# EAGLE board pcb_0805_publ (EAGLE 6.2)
DATA: 28-08-2013; WERSJA: 1.1+SMD / FINAL
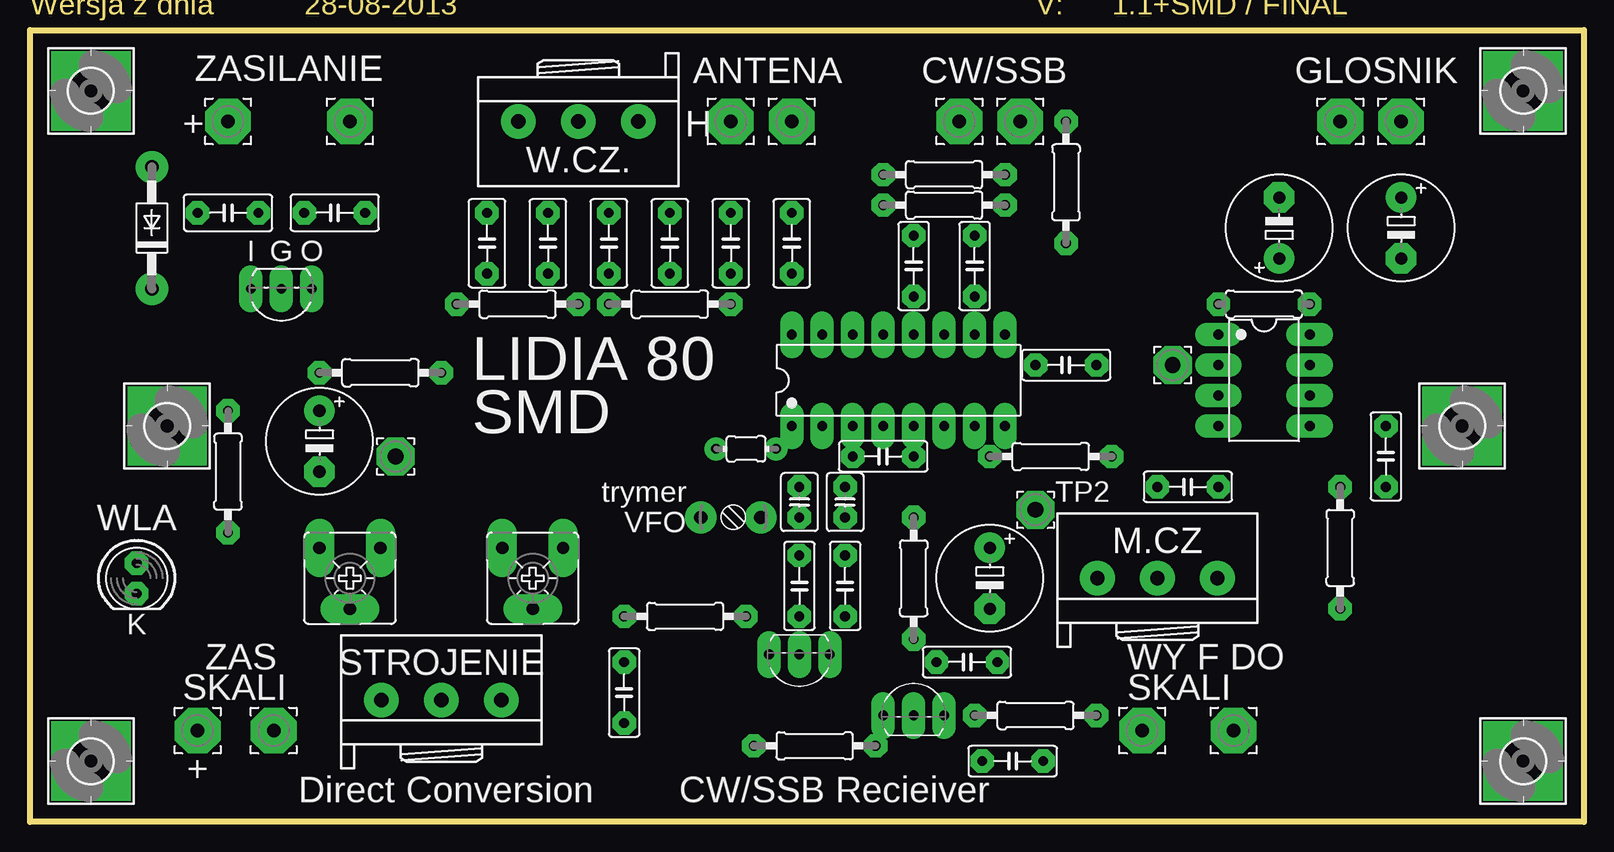
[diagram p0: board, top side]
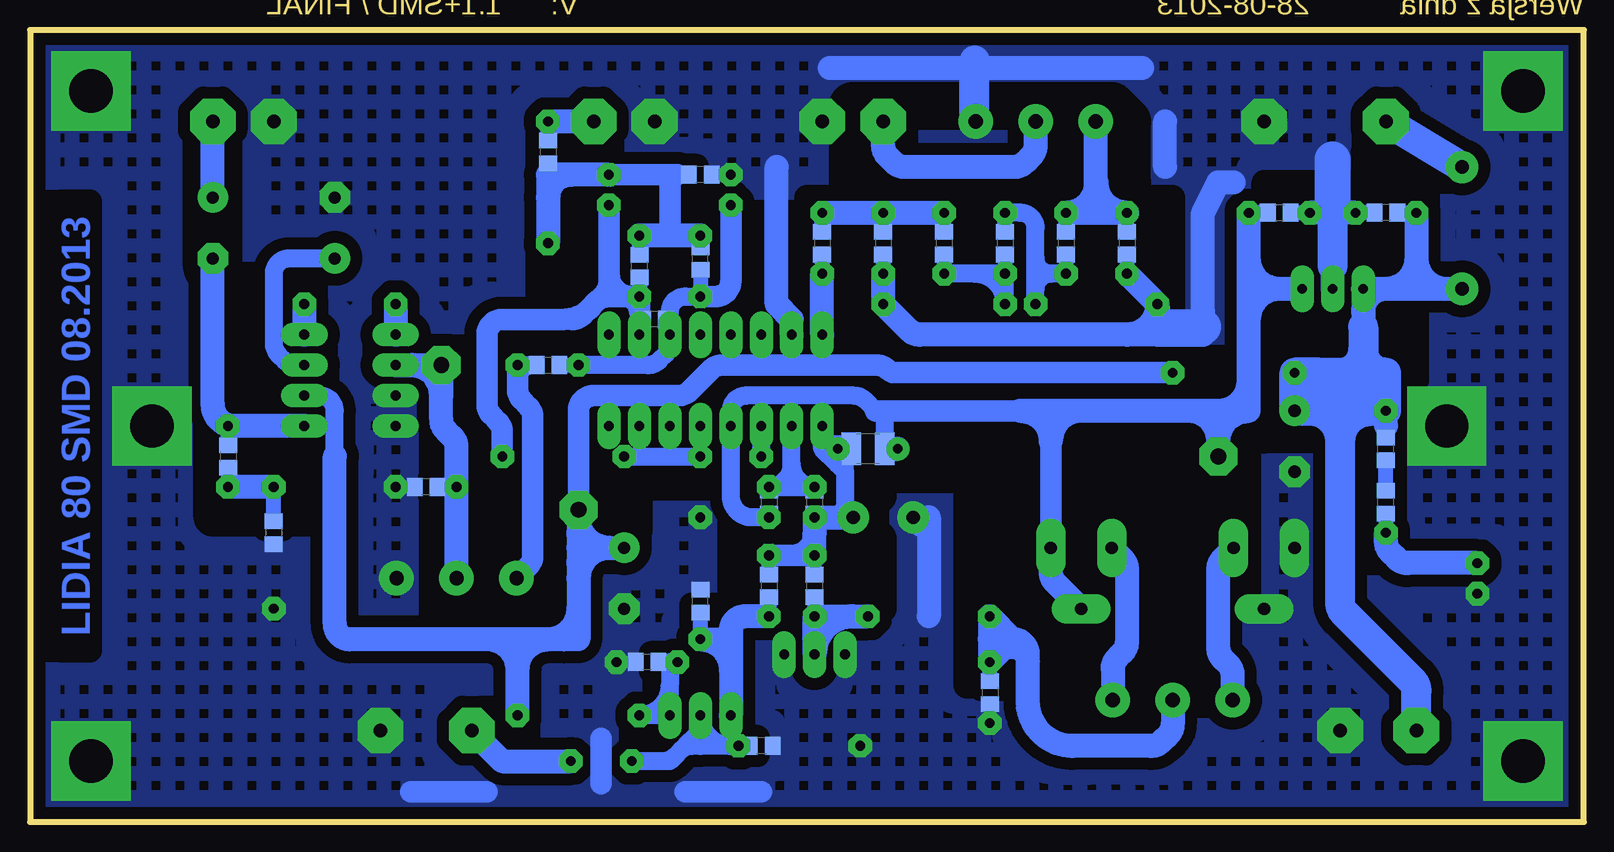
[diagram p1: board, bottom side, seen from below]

Size 129.54 x 66.04 mm. Coordinates in mm from the lower left corner, seen from the top.
Outline: 0,0 0,66.04 129.54,66.04 129.54,0 0,0
Copper layers (1*16): Top 0mil / dielectric 1.5mm / Bottom 0.035mm
Design rules: minimum track width 10mil, minimum drill 24mil, track to track 8mil, track to pad 8mil, pad to pad 8mil, via to via 8mil, smd to smd 8mil, copper to edge 5mil, drill to drill 5mil, minimum pad ring 0.1mm, minimum via ring 8mil, stop-mask expansion 10mil, vias tented up to drill 0mil, thermal gap 19mil
bRestrict: area 34.3,39.4 to 69.8,52.1; area 14,31.8 to 26.7,53.3; 28 lines

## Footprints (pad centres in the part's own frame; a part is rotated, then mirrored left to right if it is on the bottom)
3,81/1,1 = drill 1.118 pad 3.81 octagon: 1 0,0
E5-8,5 = drill 1.016 pad 2.54: + -2.54,0 | drill 1.016 pad 2.54 octagon: - 2.54,0
C050-030X075 = drill 0.813 octagon: 1 -2.54,0; 2 2.54,0
C050-025X075 = drill 0.813 octagon: 1 -2.54,0; 2 2.54,0
3050-504 = drill 1.1: 1 -2.5,0; 2 2.5,0
C025-030X050 = drill 0.813 octagon: 1 -1.27,0; 2 1.27,0
DO41-10 = drill 1.118: A 5.08,0; C -5.08,0
TO92- = drill 0.813 long: 1 2.54,0; 2 0,0; 3 -2.54,0
3,6-PAD-SQUARE = drill 3.6 pad 5.842 square: B3,6 0,0
C0805 = smd 1.3 x 1.5: 1 -0.95,0; 2 0.95,0
0207/7 = drill 0.813 octagon: 1 -3.81,0; 2 3.81,0
LAP02KR = drill 0.8 pad 1.3: 1 -2.5,0; 2 2.5,0
C1210 = smd 1.6 x 2.7: 1 -1.4,0; 2 1.4,0
0207/10 = drill 0.813 octagon: 1 -5.08,0; 2 5.08,0
LED5MM = drill 0.813 octagon: A -1.27,0; K 1.27,0
3RP/1610N = drill 1.2 pad 2.184: 1 -5,0; 2 0,0; 3 5,0
CA6V = drill 1.016 long: A -2.54,-2.54; E 2.54,-2.54; S 0,2.54
3,17/1,3 = drill 1.321 pad 3.175 octagon: 1 0,0
TO92-LINE = drill 0.813 long: 1 2.54,0; 2 0,0; 3 -2.54,0
DIL16 = drill 0.813 long: 1 -8.89,-3.81; 2 -6.35,-3.81; 3 -3.81,-3.81; 4 -1.27,-3.81; 5 1.27,-3.81; 6 3.81,-3.81; 7 6.35,-3.81; 8 8.89,-3.81; 9 8.89,3.81; 10 6.35,3.81; 11 3.81,3.81; 12 1.27,3.81; 13 -1.27,3.81; 14 -3.81,3.81; 15 -6.35,3.81; 16 -8.89,3.81
DIL08 = drill 0.813 long: 1 -3.81,-3.81; 2 -1.27,-3.81; 3 1.27,-3.81; 4 3.81,-3.81; 5 3.81,3.81; 6 1.27,3.81; 7 -1.27,3.81; 8 -3.81,3.81

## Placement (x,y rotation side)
+  [3,81/1,1]  16.51,58.42 0 top
+1  [3,81/1,1]  26.67,58.42 0 top
A_GND  [3,81/1,1]  63.5,58.42 0 top
C1  100uF  [E5-8,5]  24.13,31.75 270 top
C2  100µF  [E5-8,5]  80.01,20.32 270 top
C3  100µF  [E5-8,5]  104.14,49.53 90 top
C4  100µF  [E5-8,5]  114.3,49.53 270 top
C5  680pF  [C050-030X075]  38.1,48.26 90 top
C6  270pF  [C050-030X075]  43.18,48.26 90 top
C7  10pF  [C050-030X075]  48.26,48.26 90 top
C8  270pF  [C050-030X075]  53.34,48.26 90 top
C9  680pF  [C050-030X075]  58.42,48.26 90 top
C10  1nF  [C050-030X075]  63.5,48.26 90 top
C11  47nF  [C050-025X075]  73.66,46.35 90 top
C12  47nF  [C050-025X075]  78.74,46.35 90 top
C13  100nF  [C050-025X075]  86.36,38.1 180 top
C14  47nF  [C050-025X075]  96.52,27.94 180 top
C15  100nF  [C050-025X075]  113.03,30.48 90 top
C16  10nF  [C050-025X075]  71.12,30.48 180 top
C17  10-50pF  [3050-504]  58.42,25.4 0 top
C18  100nF  [C050-030X075]  25.4,50.8 180 top
C19  100nF  [C050-030X075]  16.51,50.8 0 top
C20  100nF  [C050-025X075]  49.53,10.79 270 top
C21  100pF  [C025-030X050]  64.14,26.67 270 top
C22  2*100pF  [C025-030X050]  67.94,26.67 270 top
C23  10nF  [C050-025X075]  64.14,19.68 270 top
C24  2,7-10pF  [C050-025X075]  67.94,19.68 270 top
C25  10nF  [C050-025X075]  81.92,5.08 0 top
C26  100nF  [C050-025X075]  78.11,13.34 0 top
CW/SSB  [3,81/1,1]  82.55,58.42 0 top
CW/SSB_GND  [3,81/1,1]  77.47,58.42 0 top
CW/SSB_GND1  [3,81/1,1]  92.71,7.62 0 top
CW/SSB_GND2  [3,81/1,1]  100.33,7.62 0 top
CW/SSB_GND3  [3,81/1,1]  20.32,7.62 0 top
CW/SSB_GND4  [3,81/1,1]  13.97,7.62 0 top
D1  1N4007  [DO41-10]  10.16,49.53 90 top
D2*  BB104G  [TO92-]  64.14,13.97 180 top
E$1  [3,6-PAD-SQUARE]  5.08,60.96 0 top
E$2  [3,6-PAD-SQUARE]  11.43,33.02 0 top
E$3  [3,6-PAD-SQUARE]  5.08,5.08 0 top
E$4  [3,6-PAD-SQUARE]  124.46,5.08 0 top
E$5  [3,6-PAD-SQUARE]  119.38,33.02 0 top
E$6  [3,6-PAD-SQUARE]  124.46,60.96 0 top
E$7  100nF  [C0805]  16.51,50.8 180 bottom
E$8  100nF  [C0805]  25.4,50.8 0 bottom
E$9  100nF  [C0805]  86.36,38.1 0 bottom
E$10  100nF  [C0805]  49.53,10.79 270 bottom
E$11  100nF  [C0805]  113.03,30.48 270 bottom
E$12  22Ω  [C0805]  109.22,24.13 270 bottom
E$13  47Ω  [C0805]  86.36,55.88 270 bottom
E$14  47Ω  [C0805]  73.66,53.98 180 bottom
E$15  gain  [0207/7]  102.87,43.18 0 top
E$16  10µH  [LAP02KR]  59.69,31.11 0 top
E$21  [ICON_PIN1_B]  63.5,34.92 0 top
E$22  [ICON_PIN1_B]  100.97,40.64 0 top
E$23  47nF  [C0805]  96.52,27.94 180 bottom
E$24  2,7-10pF  [C0805]  67.94,19.68 270 bottom
E$25  10nF  [C0805]  64.14,19.68 270 bottom
E$26  100pF  [C0805]  64.14,26.67 270 bottom
E$27  100pF  [C0805]  67.94,26.67 270 bottom
E$28  100nF  [C0805]  78.11,13.34 180 bottom
E$29  1MΩ  [C0805]  73.66,18.41 90 bottom
E$30  1kΩ  [C0805]  16.51,26.67 90 bottom
E$31  1kΩ  [C0805]  16.51,31.11 90 bottom
E$33  270pF  [C0805]  43.18,48.26 270 bottom
E$34  10pF  [C0805]  48.26,48.26 270 bottom
E$35  270pF  [C0805]  53.34,48.26 270 bottom
E$36  1nF  [C0805]  63.5,48.26 270 bottom
E$37  100kΩ  [C0805]  77.47,41.91 180 bottom
E$38  47nF  [C0805]  73.66,46.99 90 bottom
E$39  47nF  [C0805]  78.74,46.35 90 bottom
E$40  1kΩ  [C0805]  68.58,6.35 180 bottom
E$41  680pF  [C0805]  38.1,48.26 270 bottom
E$42  680pF  [C0805]  58.42,48.26 270 bottom
GLOGND  [3,81/1,1]  109.22,58.42 0 top
GLOSNIK  GLOSNIK  [3,81/1,1]  114.3,58.42 0 top
L1*  10µH  [C1210]  59.69,31.11 180 bottom
L2  10µH  [0207/10]  40.64,43.18 0 top
L3  10µH  [0207/10]  53.34,43.18 0 top
L4  100µH  [0207/10]  83.82,8.89 0 top
LED1  WLA  [LED5MM]  8.89,20.32 270 top
POT1  1kΩ  [3RP/1610N]  45.72,58.42 180 top
POT2  50kΩ  [3RP/1610N]  93.98,20.32 0 top
POT3  10kΩ  [3RP/1610N]  34.29,10.16 0 top
PR1  10kΩ  [CA6V]  26.67,20.32 180 top
PR2  10kΩ  [CA6V]  41.91,20.32 180 top
R1  2,2kΩ  [0207/10]  16.51,29.21 90 top
R2  220Ω  [0207/10]  29.21,37.47 0 top
R3  47Ω  [0207/10]  76.2,53.98 0 top
R4  100kΩ  [0207/10]  76.2,51.44 0 top
R5  47Ω  [0207/10]  86.36,53.34 90 top
R6  22Ω  [0207/10]  109.22,22.86 270 top
R7  7,5kΩ  [0207/10]  85.09,30.48 0 top
R8  100kΩ  [0207/10]  54.61,17.14 180 top
R9  1MΩ  [0207/10]  73.66,20.32 270 top
R10  1kΩ  [0207/10]  65.41,6.35 180 top
SGN  [3,81/1,1]  58.42,58.42 0 top
T1  BF245  [TO92-]  73.66,8.89 0 top
TP1  [3,17/1,3]  30.48,30.48 0 top
TP2  [3,17/1,3]  83.82,26.04 0 top
TP3  [3,17/1,3]  95.25,38.1 0 top
US1  78L08  [TO92-LINE]  20.95,44.45 180 top
US2  MC3361C  [DIL16]  72.39,36.83 0 top
US3  LM368N  [DIL08]  102.87,36.83 270 top

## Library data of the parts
+ +1 A_GND CW/SSB CW/SSB_GND CW/SSB_GND1-CW/SSB_GND4 GLOGND GLOSNIK SGN TP1-TP3 = wirepad
C1-C16 C18-C26 E$7-E$16 E$23-E$31 E$33-E$42 L1* L2-L4 R1-R10 = rcl
C17 = c-trimm
D1 = diode
D2* = transistor-npn
E$1-E$6 = holes
E$21 E$22 = dicons
LED1 = led
POT1-POT3 PR1 PR2 = pot
T1 = transistor-fet
US1 = transistor-small-signal
US2 US3 = ic-package

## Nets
GND: +1.1 A_GND.1 C1.- C2.- C3.- C5.1 C9.1 C14.1 C17.1 C18.2 C19.2 C20.2 C26.2 CW/SSB_GND2.1 CW/SSB_GND3.1 CW/SSB_GND.1 D2*.1 D2*.3 E$1.B3,6 E$2.B3,6 E$3.B3,6 E$4.B3,6 E$5.B3,6 E$6.B3,6 E$7.2 E$8.2 E$10.2 E$12.2 E$14.1 E$23.2 E$28.2 E$29.2 E$40.1 E$41.2 E$42.2 GLOGND.1 L2.1 L3.2 LED1.K POT1.1 POT2.3 PR1.E PR1.S R3.1 R6.2 R9.1 R10.2 US1.2 US2.15 US3.3 US3.4
S$1: POT1.2 SGN.1
S$2: C5.2 C6.2 E$33.1 E$41.1 POT1.3
S$3: C10.1 E$36.2 US2.16
S$4: C21.1 C22.1 US2.2
S$5: +.1 D1.A
S$6: C1.+ C19.1 CW/SSB_GND4.1 D1.C E$7.1 E$31.2 R1.2 R2.1 US1.1
S$7: C6.1 C7.2 E$33.2 E$34.1 L2.2
S$8: C8.2 C9.2 C10.2 E$35.1 E$36.1 E$42.1
S$9: C7.1 C8.1 E$34.2 E$35.2 L3.1
S$10: C11.2 C12.2 E$13.2 E$14.2 E$38.2 E$39.2 R3.2 R5.1
S$11: CW/SSB.1 E$13.1 R5.2
S$12: E$30.2 E$31.1
S$13: C11.1 C13.2 E$9.2 E$37.1 E$38.1 R4.1 US2.11
S$14: C12.1 E$37.2 E$39.1 R4.2 R7.2 US2.10
S$15: C13.1 POT2.1
S$16: C16.1 R7.1
S$17: C16.2 US2.3
S$18: C2.+ L4.2 R2.2 TP2.1 US3.6
S$19: C14.2 E$23.1 POT2.2 TP3.1 US3.2
S$20: C4.- C15.2 E$11.1 US3.5
S$21: C15.1 E$11.2 E$12.1 R6.1
S$22: E$15.2 US3.8
S$23: E$30.1 LED1.A R1.1
S$24: C4.+ GLOSNIK.1
S$25: C23.2 D2*.2 E$25.2 R8.1
S$26: C20.1 E$10.1 POT3.2 R8.2
S$27: C17.2 C21.2 C23.1 C24.1 E$16.2 E$24.1 E$25.1 L1*.2 US2.1
S$28: POT3.3 PR2.E
S$29: C3.+ US3.7
S$30: POT3.1 PR1.A
S$31: C18.1 C22.2 E$8.1 E$16.1 L1*.1 PR2.A PR2.S TP1.1 US1.3 US2.4
S$32: C25.1 E$40.2 R10.1 T1.2
S$33: C26.1 E$28.1 L4.1 T1.1
S$34: C25.2 CW/SSB_GND1.1
S$35: C24.2 E$24.2 E$29.1 R9.2 T1.3
S$36: E$15.1 US3.1

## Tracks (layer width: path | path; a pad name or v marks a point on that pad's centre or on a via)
GND
  Bottom 1.27: E$42.2 C9.1 | E$41.2 C5.1 | C18.2 E$8.2 20.95,50.8 | E$7.2 C19.2
  Bottom 1.8: 81.92,6.99 81.92,3.17 | 68.58,2.54 74.93,2.54 | 91.44,2.54 97.79,2.54
  Bottom 2: L2.1 35.56,41.27 35.56,40.64 | 35.56,40.64 38.1,40.64 | 38.1,40.64 55.35,40.64 arc45 56.25,41.01 L3.2 C9.1 | C5.1 L2.1 | US2.15 66.04,41.91 67.31,43.18 67.31,54.61 | 35.56,40.64 33.66,40.64 | 33.66,40.64 33.02,40.64 | 33.02,40.64 31.75,40.64 31.75,41.27 31.75,42.55 | 31.75,42.55 31.75,50.8 30.48,53.34 29.21,53.34 | C19.2 20.32,50.8 | 20.32,50.8 20.95,50.8 C18.2 | 20.95,50.16 arc90 20.32,50.8 | L2.1 arc-90 33.02,40.64 | L2.1 arc90 38.1,40.64 | 54.61,25.4 54.61,17.14 | 55.24,24.77 55.24,25.4 | C17.1 55.24,25.4 | 55.24,25.4 54.61,25.4 | 54.61,25.4 arc-90 55.24,24.77 | 55.24,24.77 arc90 54.61,25.4 | 33.66,40.64 arc-90 31.75,42.55 | 34.92,54.61 34.92,58.42 | 36.83,62.87 62.87,62.87 | US1.2 20.95,46.35
  Bottom 2.5: POT1.1 arc90 50.8,58.5 50.8,63.5 | 20.95,46.35 20.95,50.8
  Bottom 3: 20.95,50.8 20.95,55.24 | 35.56,41.27 31.75,41.27
  pour Bottom (isolate 1, no thermals, hatched): 129.54,0 0,0 0,66.04 129.54,66.04
S$1
  Bottom 2: POT1.2 45.72,56.41 arc45 46.09,55.51 46.62,54.98 arc45 47.52,54.61 56.62,54.61 arc45 57.52,54.98 58.05,55.51 arc45 58.42,56.41 SGN.1
S$2
  Bottom 1.27: E$33.1 C6.2 | E$41.1 C5.2
  Bottom 1.5: 40.72,50.88 40.64,50.8
  Bottom 2: POT1.3 40.72,50.88 | C6.2 40.64,50.8 C5.2 arc90 40.64,53.34 arc90 C6.2
S$3
  Bottom 1.27: E$36.2 C10.1
  Bottom 2: US2.16 C10.1
S$4
  Bottom 1.5: 65.41,27.94 66.04,27.94 66.04,29.84 | 66.04,29.84 US2.2 | 66.04,29.84 arc-90 C21.1 C22.1 arc-90 66.04,29.84
S$5
  Bottom 2.54: +.1 D1.A
S$6
  Bottom 1.27: E$31.2 16.51,33.02 | E$7.1 C19.1
  Bottom 2: 16.51,33.02 R1.2 | D1.C 11.43,44.45 | 11.43,44.45 13.97,44.45 | 16.51,44.45 US1.1 18.41,42.55 | C19.1 13.97,46.99 | 13.97,46.99 13.97,44.45 | 18.41,42.55 18.41,41.27 | 13.97,44.45 16.51,44.45 | 16.51,44.45 arc-90 18.41,42.55 | 13.97,46.99 arc90 16.51,44.45 | 13.97,46.99 arc-90 11.43,44.45
  Bottom 2.5: 24.13,35.56 R2.1 22.23,37.47 | 22.23,37.47 20.32,37.47 | 20.32,37.47 19.05,37.47 | 19.05,37.47 18.41,37.47 | 18.41,37.47 16.51,37.47 | 16.51,37.47 R1.2 | 18.41,41.27 18.41,39.37 | 18.41,39.37 18.41,37.47 | R1.2 16.51,34.92 arc-90 19.05,37.47 | 16.51,37.47 arc90 18.41,39.37 | 20.32,37.47 arc-90 18.41,39.37 | 24.13,35.56 arc90 22.23,37.47 | CW/SSB_GND4.1 13.97,10.9 arc-45 14.34,11.8 19.95,17.41 arc45 20.32,18.31 20.32,31.75 | 20.32,31.75 20.32,35.56 | 20.32,35.56 20.32,37.47 | 20.32,35.56 arc90 18.41,37.47 | 20.32,35.56 arc-90 22.23,37.47 | R1.2 17.78,34.29 | 17.78,34.29 22.86,34.29 | 22.86,34.29 C1.+ 24.13,35.56 | 24.13,35.56 19.05,35.56 | 20.32,31.75 arc90 17.78,34.29 | 20.32,31.75 arc-90 22.86,34.29
S$7
  Bottom 1.27: E$33.2 C6.1 | E$34.1 C7.2
  Bottom 1.5: L2.2 45.72,44.45 | 45.72,44.45 45.72,45.72 | 45.72,45.72 45.72,46.99 | 45.72,45.72 C6.1 44.45,45.72 | 44.45,45.72 arc90 45.72,46.99 | 44.45,45.72 arc-90 45.72,44.45 | 45.72,46.99 45.72,49.53 arc-90 46.99,50.8 C7.2
S$8
  Bottom 1.27: E$35.1 C8.2 | E$36.1 C10.2 | E$42.1 C9.2
  Bottom 2: C10.2 C9.2 C8.2
S$9
  Bottom 1.27: E$34.2 C7.1 | E$35.2 C8.1
  Bottom 1.5: 50.8,45.72 C7.1 L3.1 arc-90 50.8,45.72 | 50.8,45.72 C8.1
S$10
  Bottom 1.27: 75.56,53.98 E$14.2 | E$38.2 C11.2 | E$39.2 C12.2
  Bottom 1.3: E$13.2 86.36,53.98
  Bottom 1.8: R3.2 76.2,53.98 | 76.2,53.98 75.56,53.98 | 76.2,48.9 76.2,53.98
  Bottom 2: R3.2 84.45,53.98 | 84.45,53.98 86.36,53.98 86.36,52.07 | 86.36,52.07 R5.1 | 84.45,53.98 arc-90 86.36,52.07 | C12.2 76.2,48.9 C11.2
S$11
  Bottom 1.3: E$13.1 R5.2
  Bottom 2: R5.2 CW/SSB.1
S$12
  Bottom 1.27: E$30.2 E$31.1
S$13
  Bottom 1.27: E$9.2 C13.2 | E$38.1 C11.1 | 76.2,42.55 76.2,42.23 arc90 E$37.1
  Bottom 1.5: C13.2 78,38.1 arc-45 77.1,38.47 76.57,39 arc-45 76.2,39.9 US2.11 76.2,42.55 arc90 74.93,43.81 C11.1
  Bottom 1.8: R4.1 71.12,45.09 arc90 72.39,43.81 C11.1
S$14
  Bottom 1.27: E$37.2 78.74,41.91 | E$39.1 78.74,44.45 79.38,43.81
  Bottom 1.5: US2.10 78.74,41.91 78.74,42.55 | 85.09,41.91 84.35,41.91 | 80.64,43.81 81.28,44.45 | 81.28,44.45 81.28,44.98 | 81.65,44.08 81.28,44.45 | 80.01,43.81 79.38,43.81
  Bottom 1.8: R7.2 90.17,32.49 arc-45 90.54,33.39 91.07,33.92 arc45 91.44,34.82 91.44,40.64 arc90 90.17,41.91 85.09,41.91 arc-53 82.55,43.18 | 84.35,41.91 arc-45 83.45,42.28 82.55,43.18 | 81.28,45.72 R4.2 | 82.55,43.18 arc53 81.28,43.81 80.01,43.81 arc90 78.74,42.55 C12.1 79.38,43.81 arc90 81.28,45.72 | 81.28,45.72 81.28,44.98 arc45 81.65,44.08 82.55,43.18
S$15
  Bottom 1.5: 88.9,36.83 arc90 87.63,38.1 C13.1
  Bottom 1.8: C13.1 88.9,36.83 88.9,36.09 arc-45 88.53,35.19 88,34.66 arc45 87.63,33.76 87.63,22.2 arc45 88,21.3 POT2.1
S$16
  Bottom 1.5: R7.1 C16.1
S$17
  Bottom 1.5: C16.2 US2.3
S$18
  Bottom 1.5: 104.14,30.48 104.14,34.29 arc-90 105.41,35.56 US3.6
  Bottom 1.8: TP2.1 83.82,34.29 arc90 82.55,35.56 75.46,35.56 arc-45 74.56,35.93 72.76,37.73 arc45 71.86,38.1 58.95,38.1 arc45 58.05,37.73 arc-45 57.41,37.47 R2.2
  Bottom 2: 83.82,22.86 83.82,21.59 | 83.82,21.59 83.82,20.32 | 83.82,20.32 83.82,17.78 | 83.82,17.78 83.82,16.51 | 83.82,16.51 83.82,15.24 85.09,15.24 | 83.82,25.4 83.82,24.13 | 83.82,22.86 82.55,22.86 | 85.09,15.24 86.36,15.24 | 86.36,15.24 88.9,15.24 | 88.9,15.24 91.44,15.24 | 91.44,15.24 102.87,15.24 arc90 104.14,16.51 104.14,30.48 | 82.55,22.86 arc90 83.82,24.13 | 83.82,24.13 83.82,22.86 | 83.82,21.59 arc90 82.55,22.86 | 85.09,15.24 arc-90 83.82,16.51 | 86.36,15.24 arc-90 83.82,17.78 | 83.82,25.4 arc-90 81.28,22.86 arc-90 83.82,20.32 | 82.55,22.86 C2.+ | 83.82,25.4 TP2.1 | L4.2 88.9,11.43 88.9,12.7 | 88.9,12.7 88.9,15.24 | 88.9,12.7 arc90 86.36,15.24 | 88.9,12.7 arc-90 91.44,15.24
S$19
  Bottom 0.406: E$23.1 C14.2
  Bottom 2: POT2.2 C14.2 93.98,31.22 arc-45 94.35,32.12 94.88,32.65 arc45 95.25,33.55 95.25,35.56 | US3.2 97.79,38.1 | 95.25,35.56 TP3.1 97.79,38.1 | 95.25,35.56 arc-90 97.79,38.1
S$20
  Bottom 1: E$11.1 113.03,31.75
  Bottom 1.27: 113.03,31.75 C15.2
  Bottom 2: US3.5 C15.2 112.53,33.02 arc90 114.3,34.79 C4.-
S$21
  Bottom 1.27: E$11.2 C15.1 | E$12.1 R6.1
  Bottom 2: R6.1 C15.1
S$22
  Bottom 2: E$15.2 US3.8
S$23
  Bottom 1.27: E$30.1 R1.1
  Bottom 2: LED1.A 14.71,21.59 arc45 15.61,21.96 16.14,22.49 arc45 16.51,23.39 R1.1
S$24
  Bottom 2: C4.+ GLOSNIK.1
S$25
  Bottom 1.27: E$25.2 C23.2
  Bottom 2: 60.96,17.14 C23.2 D2*.2 arc90 60.96,17.14 | 60.96,17.14 R8.1
S$26
  Bottom 1.27: E$10.1 C20.1
  Bottom 2: POT3.2 34.29,8.15 arc45 34.66,7.25 35.19,6.72 arc45 36.09,6.35 42.65,6.35 arc90 46.35,10.05 46.35,13.34 | 46.35,13.34 46.35,13.97 arc-90 47.62,15.24 | 47.62,15.24 49.53,15.24 | 49.53,15.24 R8.2 47.62,15.24 | 49.53,15.24 C20.1 47.62,15.24 | 48.9,14.61 47.62,14.61 arc90 46.35,13.34
S$27
  Bottom 1: 63.5,31.75 60.96,31.75
  Bottom 1.27: E$24.1 C24.1 | E$25.1 C23.1
  Bottom 1.5: 60.96,25.5 arc-45 C17.2 | 63.5,31.75 arc-90 62.87,31.11 62.23,31.11 62.23,29.84 | 63.5,31.75 US2.1 | L1*.2 E$16.2 | 61.59,29.21 61.59,26.56 arc45 61.97,25.66 62.23,25.4 | 61.59,29.21 62.23,29.84 | 62.23,29.84 63.5,31.11 63.5,31.75 | 61.59,29.21 61.59,30.48
  Bottom 1.8: C23.1 66.04,22.23 | 66.04,22.23 C24.1 | 64.14,24.13 arc90 66.04,22.23
  Bottom 2: 60.96,25.44 C17.2 62.23,25.4 C21.2 64.14,24.13 C23.1 | 62.23,31.11 E$16.2
S$28
  Bottom 2: POT3.3 39.29,12.78 arc45 38.92,13.68 38.47,14.12 arc-45 38.1,15.02 38.1,21.06 arc-45 38.47,21.96 PR2.E
S$29
  Bottom 1.5: US3.7 107.42,38.1 arc45 108.32,38.47 108.85,39 arc45 109.22,39.9 109.22,45.72 arc90 107.95,46.99 C3.+
S$30
  Bottom 2: POT3.1 29.29,12.25 arc-45 29.66,13.15 30.11,13.6 arc45 30.48,14.5 30.48,21.06 arc45 30.11,21.96 PR1.A
S$31
  Bottom 1.27: E$8.1 C18.1
  Bottom 1.5: 58.92,34.42 58.29,34.29 L1*.1 57.78,31.11 | C22.2 69.32,25.4 arc90 71.12,27.2 US2.4 71.12,34.29 arc90 69.85,35.56 60.85,35.56 arc45 59.95,35.19 59.05,34.29
  Bottom 1.8: 46.99,34.29 58.29,34.29 59.05,34.29 | PR2.A 44.45,31.75 44.45,34.29
  Bottom 2: PR2.S 44.08,19.95 arc45 44.45,20.85 PR2.A | 27.94,34.29 27.94,36.83 | 27.94,34.29 30.48,34.29 | 30.48,34.29 33.02,34.29 | 33.02,34.29 41.91,34.29 | 41.91,34.29 44.45,34.29 46.99,34.29 arc90 44.45,31.75 arc90 41.91,34.29 | 30.48,34.29 arc-90 27.94,36.83 | 27.94,36.83 27.94,41.91 | 27.94,41.91 27.94,44.45 | 27.94,44.45 27.94,46.99 | 27.94,46.99 C18.1 | US1.3 25.4,44.45 | 25.4,44.45 27.94,44.45 | 25.4,44.45 arc90 27.94,46.99 | 25.4,44.45 arc-90 27.94,41.91 | 57.78,31.11 E$16.1 | TP1.1 30.48,31.75 | 30.48,31.75 30.48,34.29 | 30.48,31.75 arc90 27.94,34.29 | 30.48,31.75 arc-90 33.02,34.29
S$32
  Bottom 1.27: E$40.2 R10.1
  Bottom 1.5: R10.1 71.12,6.35 | 71.12,6.35 73.66,6.35 | 74.4,6.35 arc-45 75.3,5.98 | 75.3,5.98 75.83,5.45 | 75.83,5.45 arc45 76.73,5.08 | 76.73,5.08 C25.1 | T1.2 73.66,6.35 | T1.2 arc-90 71.12,6.35 | T1.2 73.66,7.62 arc90 74.93,6.35 74.03,7.25 arc-45 73.66,8.15 T1.2 | 73.66,6.35 74.4,6.35 | 74.4,6.35 arc-45 75.3,5.98 | 75.83,5.45 76.2,5.08 76.73,5.08
S$33
  Bottom 1.27: E$28.1 C26.1
  Bottom 1.5: 76.2,10.9 T1.1 L4.1 arc-90 76.2,11.43 76.2,13.34 C26.1
S$34
  Bottom 2: CW/SSB_GND1.1 90.17,5.08 C25.2
S$35
  Bottom 1.27: E$24.2 C24.2 | R9.2 E$29.1
  Bottom 2: C24.2 69.96,17.14 arc-90 71.12,15.98 71.12,15.24 | 71.12,15.24 71.12,12.7 | 71.12,12.7 T1.3 | 71.12,15.24 R9.2 arc90 71.12,12.7
S$36
  Bottom 2: E$15.1 US3.1

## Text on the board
Bottom: LIDIA 80 SMD 08.2013
Dimension: Wersja z dnia | V:
tPlace: ZASILANIE | ANTENA | + | H | W.CZ. | I | G | O | LIDIA 80 | SMD | trymer | VFO | M.CZ | K | ZAS | STROJENIE | WY F DO | SKALI | SKALI | + | Direct Conversion | CW/SSB Recieiver
tValues: +
Document: A | B | C | D | 1 | 2 | 3 | 4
